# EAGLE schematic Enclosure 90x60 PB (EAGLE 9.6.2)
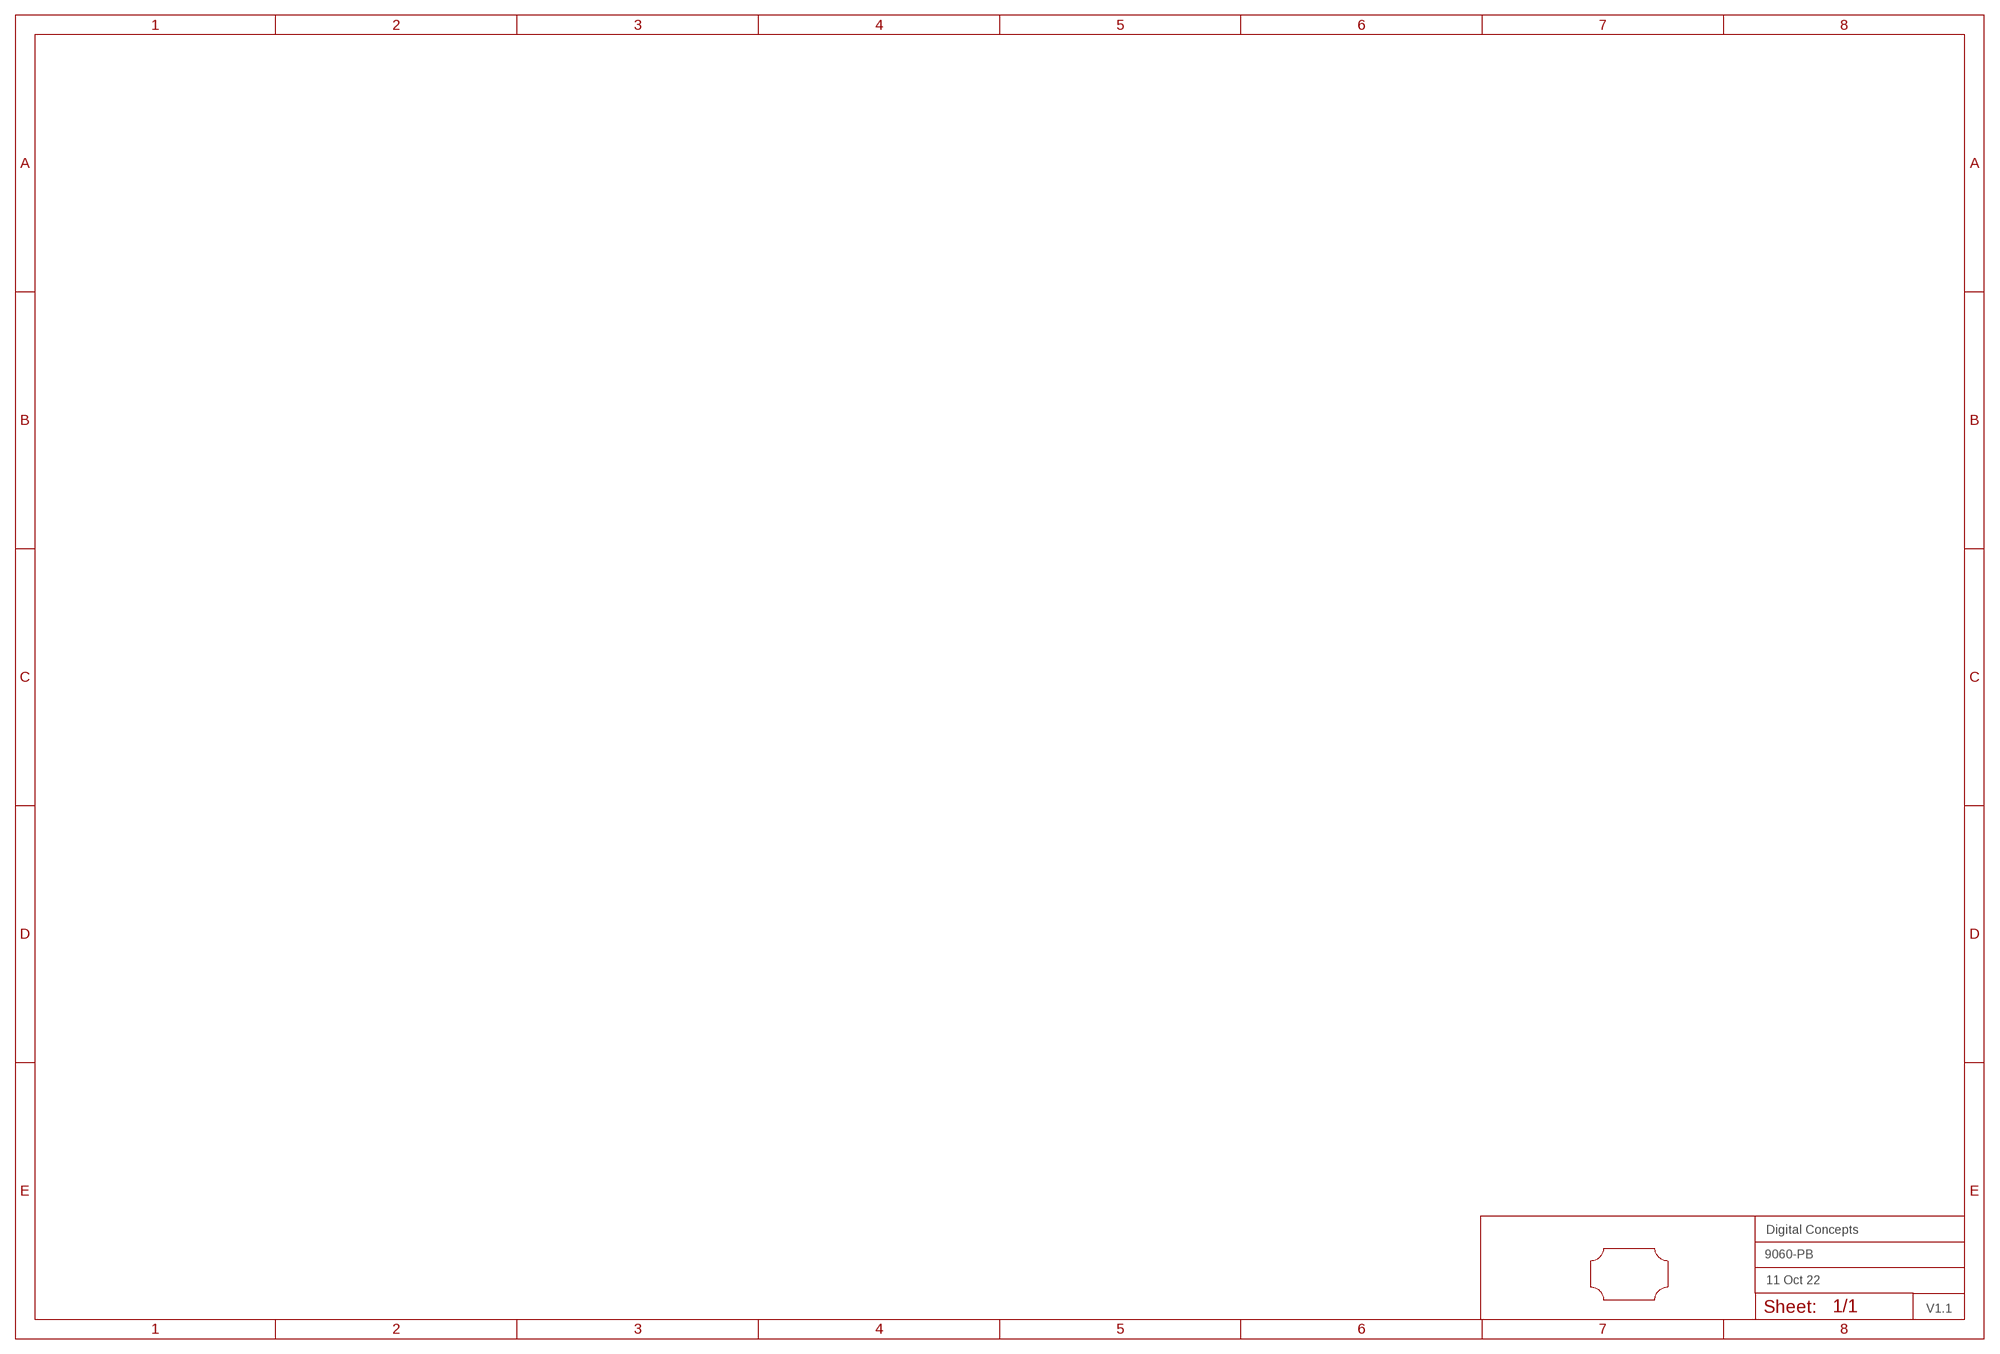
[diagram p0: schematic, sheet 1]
FRAME2 (A3L-LOC): DATE: 11 Oct 22; OWNER: Digital Concepts; TITLE: 9060-PB; VERSION: V1.1

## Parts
U$1  PROTO-32X21  [PROTO-90X60]

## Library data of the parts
U$1 = digitalconcepts:PROTO-32X21: Prototyping board with 32x21 pad matrix for 90 x 60 enclosure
